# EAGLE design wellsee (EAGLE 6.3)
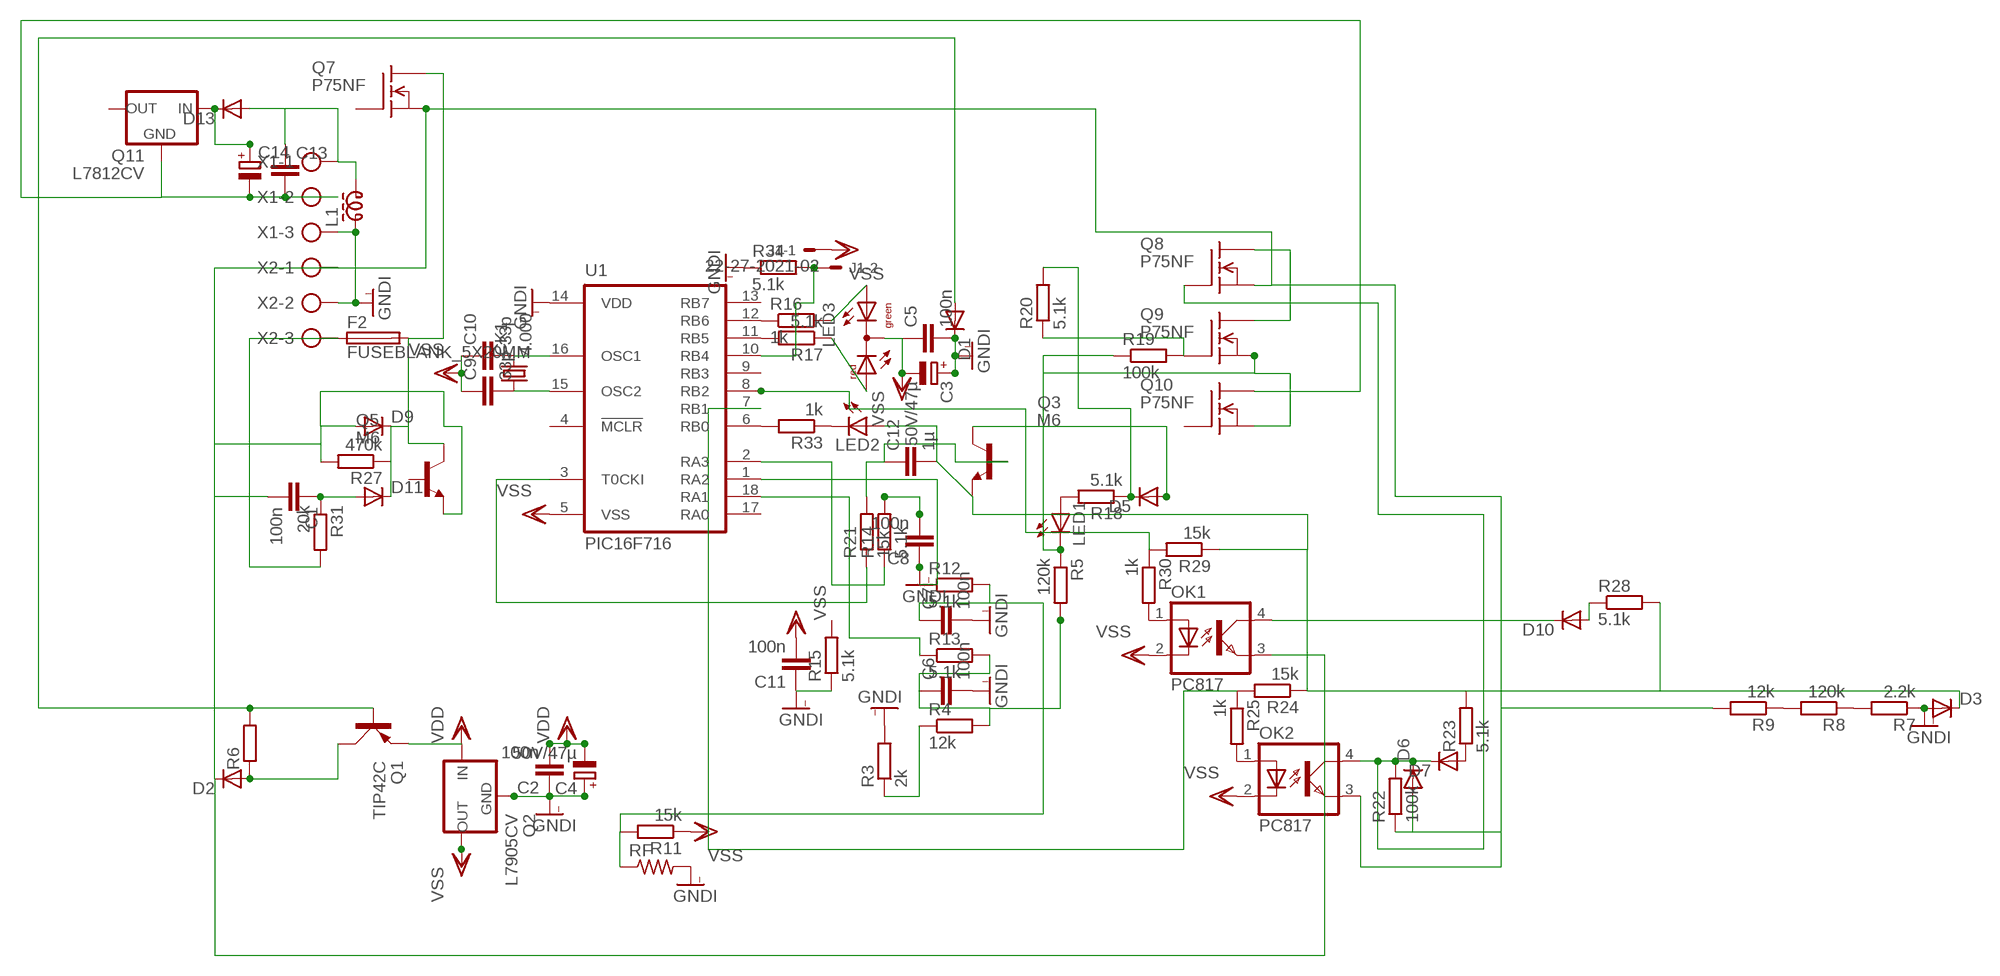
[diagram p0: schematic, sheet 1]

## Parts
C1  100n  C-EUC0805  [C0805]
C2  100n  C-EUC0805  [C0805]
C3  50V/47µ  CPOL-EUE2.5-6  [E2,5-6]
C4  50V/47µ  CPOL-EUE2.5-6  [E2,5-6]
C5  100n  C-EUC0805  [C0805]
C6  100n  C-EUC0805  [C0805]
C7  100n  C-EUC0805  [C0805]
C8  100n  C-EUC0805  [C0805]
C9  33p  C-EUC0805  [C0805]
C10  33p  C-EUC0805  [C0805]
C11  100n  C-EUC0805  [C0805]
C12  1µ  C-EUC0805  [C0805]
C13  C-EU075-032X103  [C075-032X103]
C14  CPOL-EUE5-13  [E5-13]
CK1  4.000  CRYSTALHC49S  [HC49/S]
D1  DIODE-MINIMELF  [MINIMELF]
D2  DIODE-MINIMELF  [MINIMELF]
D3  DIODE-MELF-MLL41  [MELF-MLL41]
D5  DIODE-MINIMELF  [MINIMELF]
D6  DIODE-MINIMELF  [MINIMELF]
D7  DIODE-MINIMELF  [MINIMELF]
D9  DIODE-MINIMELF  [MINIMELF]
D10  DIODE-MINIMELF  [MINIMELF]
D11  DIODE-MELF-MLL41  [MELF-MLL41]
D13  DIODE-MELF-MLL41  [MELF-MLL41]
F2  FUSEBLANK_5X20MM  [FUSE_HOLDER_5X20MM]
J1  22-27-2021-02  [6410-02]
L1  ZD60820512  [ZD6-2W5]
LED1  LED3MM  [LED3MM]
LED2  LED3MM  [LED3MM]
LED3  DUOLED-RG-C  [DUOLED-C-5MM]
OK1  PC817  [DIL04]
OK2  PC817  [DIL04]
Q1  TIP42C  [TO220AV]
Q2  L7905CV  79XXS  [79XXS]
Q3  M6  BC849SMD  [SOT23-BEC]
Q5  M6  BC849SMD  [SOT23-BEC]
Q7  P75NF  SUP75N06-08  [TO220]
Q8  P75NF  SUP75N06-08  [TO220]
Q9  P75NF  SUP75N06-08  [TO220]
Q10  P75NF  SUP75N06-08  [TO220]
Q11  L7812CV  78XXS  [78XXS]
R3  2k  R-EU_R0805  [R0805]
R4  12k  R-EU_R0805  [R0805]
R5  120k  R-EU_R0805  [R0805]
R6  R-EU_0207/5V  [0207/5V]
R7  2.2k  R-EU_R0805  [R0805]
R8  120k  R-EU_R0805  [R0805]
R9  12k  R-EU_R0805  [R0805]
R11  15k  R-EU_R0805  [R0805]
R12  5.1k  R-EU_R0805  [R0805]
R13  5.1k  R-EU_R0805  [R0805]
R14  5.1k  R-EU_R0805  [R0805]
R15  5.1k  R-EU_R0805  [R0805]
R16  1k  R-EU_R0805  [R0805]
R17  5.1k  R-EU_R0805  [R0805]
R18  5.1k  R-EU_R0805  [R0805]
R19  100k  R-EU_R0805  [R0805]
R20  5.1k  R-EU_R0805  [R0805]
R21  15k  R-EU_R0805  [R0805]
R22  100k  R-EU_R0805  [R0805]
R23  5.1k  R-EU_R0805  [R0805]
R24  15k  R-EU_R0805  [R0805]
R25  1k  R-EU_R0805  [R0805]
R27  470k  R-EU_R0805  [R0805]
R28  5.1k  R-EU_R0805  [R0805]
R29  15k  R-EU_R0805  [R0805]
R30  1k  R-EU_R0805  [R0805]
R31  20k  R-EU_R0805  [R0805]
R33  1k  R-EU_R0805  [R0805]
R34  5.1k  R-EU_R0805  [R0805]
RF  R-US_0204/2V  [0204V]
U1  PIC16F716  PIC16C52JW  [DIL18]
X1  AK500/3  [AK500/3]
X2  AK500/3  [AK500/3]

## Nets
GNDI: C2.1 C3.+ C4.+ C5.2 C6.2 C7.2 C8.1 C11.1 D1.C D3.A L1.1 Q2.GND R3.2 R7.1 R15.1 R34.1 RF.2 U1.14(VDD) X1.3 X2.2
N$1: C9.2 CK1.1 U1.15(OSC2)
N$2: C10.2 CK1.2 U1.16(OSC1)
N$3: C7.1 R11.2 R12.2 RF.1
N$5: R33.2 U1.6(RB0)
N$6: LED2.K(C) R33.1
N$7: LED3.AR R17.1
N$8: LED3.AX(AG) R16.2
N$9: R16.1 U1.12(RB6)
N$10: R17.2 U1.11(RB5)
N$11: J1.2 R34.2 U1.10(RB4)
N$12: R14.1 U1.2(RA3)
N$13: R3.1 R4.1
N$14: C6.1 R4.2 R5.2 R13.2
N$15: R13.1 U1.18(RA1)
N$16: LED1.K(C) Q9.3(S) Q10.3(S) R5.1 R19.1
N$17: R21.1 U1.3(T0CKI)
N$18: R12.1 U1.1(RA2)
N$19: C8.2 R14.2
N$20: C12.1 Q3.B R21.2
N$21: C1.2 D2.C D6.A D9.A OK1.3(EMIT) OK2.3(EMIT) Q5.E Q7.3(S) Q8.3(S) R9.2 R22.1 R27.2 X2.1
N$22: C12.2 D3.C LED2.A Q3.E R23.2 R24.1 R28.2 R29.1
N$25: R29.2 R30.1 U1.8(RB2)
N$26: D5.C R18.1 R20.2
N$27: D5.A Q3.C
N$28: OK1.1(A) R30.2
N$29: OK2.1(A) R25.2
N$30: R24.2 R25.1 U1.7(RB1)
N$31: LED1.A R18.2
N$32: D6.C D7.C OK2.4(COL) Q8.1(G) R22.2
N$33: D7.A R23.1
N$34: R8.2 R9.1
N$35: R7.2 R8.1
N$36: Q8.2(D) Q9.2(D)
N$37: D10.C OK1.4(COL)
N$38: D1.A Q1.B R6.2
N$39: D10.A R28.1
N$40: D2.A Q1.C R6.1
N$44: Q9.1(G) R19.2 R20.1
N$48: F2.1 R31.2 X2.3
N$49: D9.C D11.C F2.2 Q5.C Q7.2(D) R27.1
N$51: C13.1 D13.A L1.2 X1.1
N$54: C14.+ D13.C Q11.IN
N$55: C13.2 C14.- Q10.2(D) Q11.GND X1.2
N$56: C1.1 D11.A R31.1
VDD: C2.2 C4.- Q1.E Q2.IN
VSS: C3.- C5.1 C9.1 C10.1 C11.2 J1.1 LED3.C OK1.2(C) OK2.2(C) Q2.OUT R11.1 U1.5(VSS)
Unconnected: Q5.B Q7.1(G) Q10.1(G) Q11.OUT R15.2 U1.4(!MCLR) U1.9(RB3) U1.13(RB7) U1.17(RA0)

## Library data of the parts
C1 C2 C5-C13 = rcl:C-EU: CAPACITOR, European symbol
C3 C4 C14 = rcl:CPOL-EU: POLARIZED CAPACITOR, European symbol
CK1 = crystal:CRYSTAL: CRYSTAL; OC_FARNELL: 1667008; OC_NEWARK: unknown
D1-D3 D5-D7 D9-D11 D13 = diode:DIODE-: DIODE
F2 = fuse:FUSE: Fuse; OC_FARNELL: unknown; OC_NEWARK: unknown
J1 = con-molex:22-?-02: CONNECTOR; OC_FARNELL: unknown; OC_NEWARK: unknown
L1 = inductor-neosid:ZD60820512: WIDE-BAND CHOKE; OC_FARNELL: unknown; OC_NEWARK: unknown
LED1 LED2 = led:LED: LED
LED3 = led:DUOLED-RG-C: DUO LED 2 colors (red/green), 5 mm, round, common Cathode www.ligitek.com or other producers.
OK1 OK2 = optocoupler:PC817: SHARP OPTO COUPLER; MPN: PC817X4J000F; OC_FARNELL: 9707727; OC_NEWARK: 97K7059
Q1 = transistor-power:TIP42C: PNP TRANSISTOR
Q2 = v-reg:79XXS: VOLTAGE REGULATOR
Q3 Q5 = transistor-npn:BC849*: NPN Transistor
Q7-Q10 = transistor-fet:SUP75N06-08: N-Channel Enhancement MOSFET 60V; 75A; 0,008Ohm
Q11 = v-reg:78XXS: VOLTAGE REGULATOR
R3-R9 R11-R25 R27-R31 R33 R34 = rcl:R-EU_: RESISTOR, European symbol
RF = rcl:R-US_: RESISTOR, American symbol
U1 = microchip:PIC16C52: MICROCONTROLLER; OC_FARNELL: unknown; OC_NEWARK: unknown
X1 X2 = con-ptr500:AK500/3: CONNECTOR; OC_FARNELL: unknown; OC_NEWARK: unknown

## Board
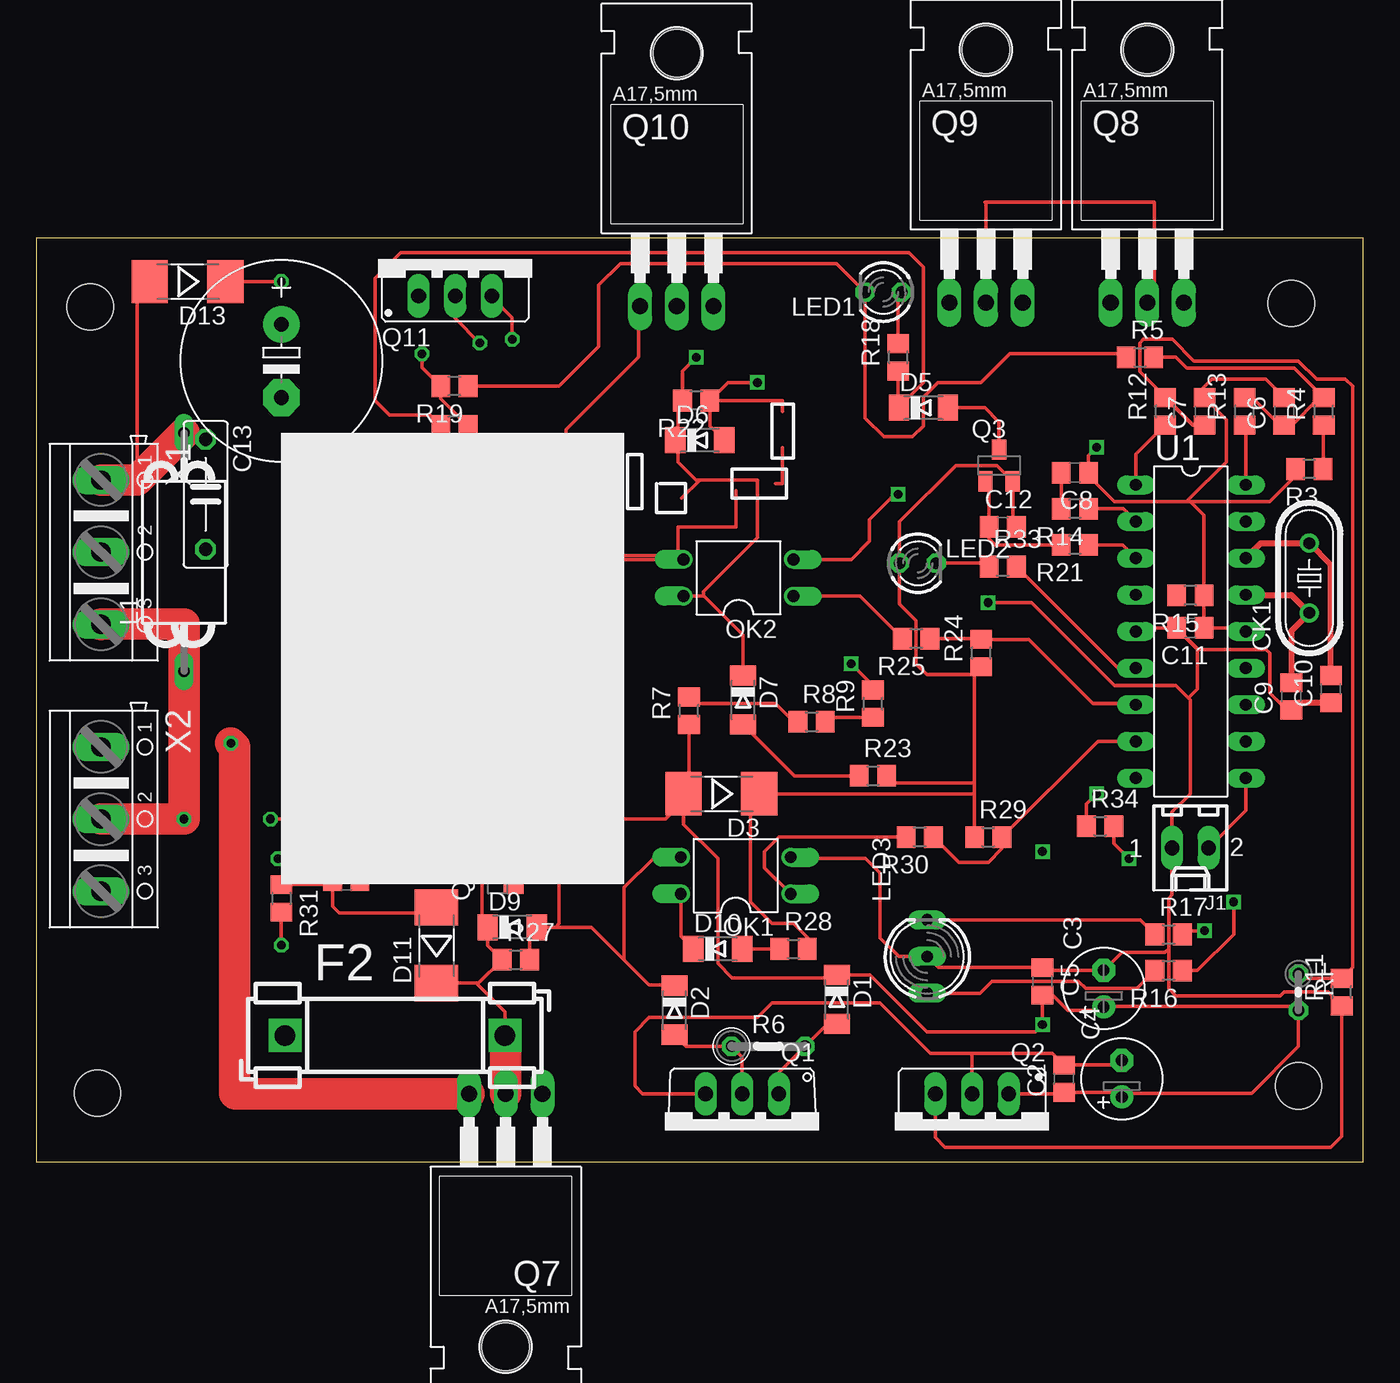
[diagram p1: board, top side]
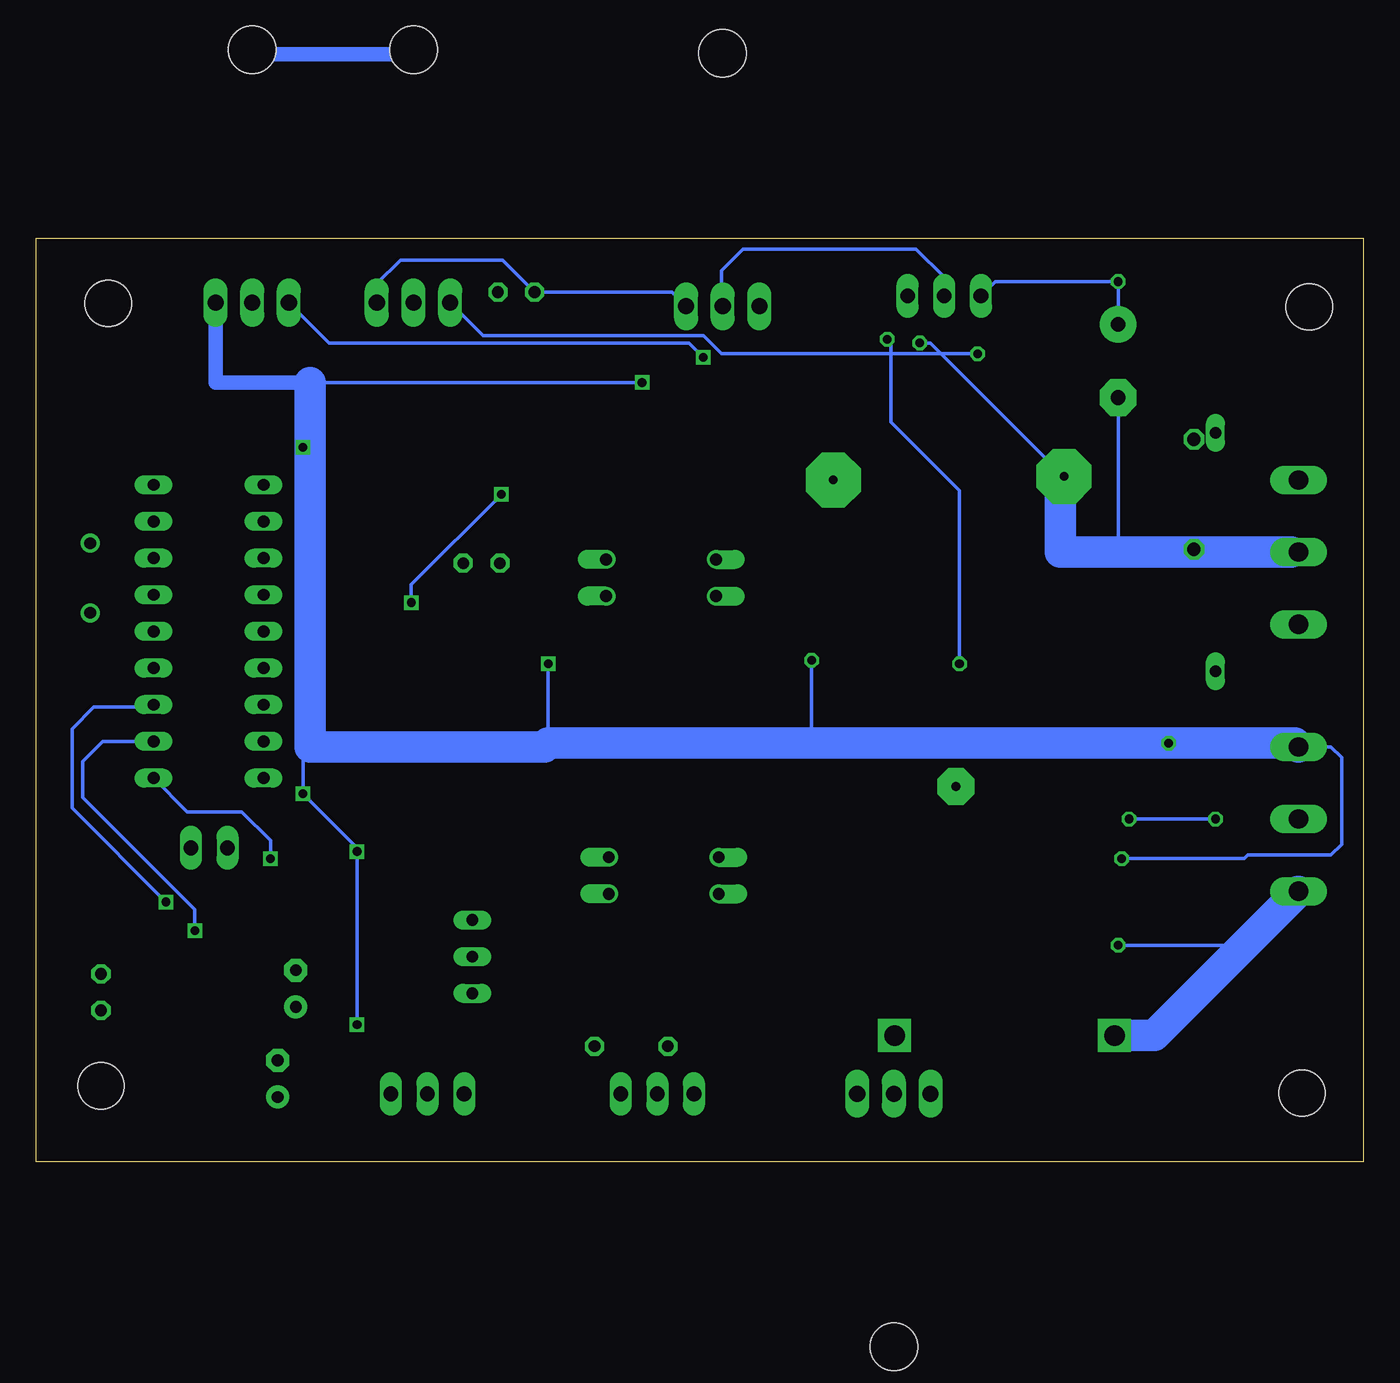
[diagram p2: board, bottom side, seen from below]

Size 92 x 64 mm. Coordinates in mm from the lower left corner, seen from the top.
Outline: 0,0 92,0 92,64 0,64 0,0
Copper layers (1*16): Top 0.035mm / dielectric 1.5mm / Bottom 0.035mm
Design rules "default": minimum track width 10mil, minimum drill 24mil, track to track 8mil, track to pad 8mil, pad to pad 8mil, via to via 8mil, smd to smd 8mil, copper to edge 40mil, drill to drill 8mil, minimum pad ring 10mil, minimum via ring 8mil, stop-mask expansion 4mil, vias tented up to drill 0mil, thermal gap 10mil
Holes 3.2 mm at 3.75,59.25 87,59.5 87.5,5.25 4.25,4.75

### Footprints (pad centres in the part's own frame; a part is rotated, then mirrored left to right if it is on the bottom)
C0805 = smd 1.3 x 1.5: 1 -0.95,0; 2 0.95,0
E2,5-6 = drill 0.813 pad 1.6: + -1.27,0 | drill 0.813 pad 1.6 octagon: - 1.27,0
C075-032X103 = drill 0.914 octagon: 1 -3.81,0; 2 3.81,0
E5-13 = drill 1.016 pad 2.54: + -2.54,0 | drill 1.016 pad 2.54 octagon: - 2.54,0
HC49/S = drill 0.813: 1 -2.413,0; 2 2.413,0
MINIMELF = smd 1.4 x 1.8: A 1.7,0; C -1.7,0
MELF-MLL41 = smd 2.5 x 3: A 2.625,0; C -2.625,0
FUSE_HOLDER_5X20MM = drill 1.422 pad 2.286 square: 1 0,0; 2 15.24,0
6410-02 = drill 1.016 long: 1 1.27,0; 2 -1.27,0
ZD6-2W5 = drill 0.8 long: 1 -8.255,0; 2 8.255,0
LED3MM = drill 0.813 octagon: A -1.27,0; K 1.27,0
DUOLED-C-5MM = drill 0.813 long: AR 2.54,0; AX -2.54,0; C 0,0
DIL04 = drill 0.813 offset: 1 -1.27,-3.81; 2 1.27,-3.81; 3 1.27,3.81; 4 -1.27,3.81
TO220AV = drill 1.016 long: B -2.54,-2.54; C 0,-2.54; E 2.54,-2.54
79XXS = drill 1.016 long: GND -2.54,-2.54; IN 0,-2.54; OUT 2.54,-2.54
SOT23-BEC = smd 1 x 1.4: B -0.95,-1.1; C 0,1.1; E 0.95,-1.1
TO220 = drill 1.118 long: 1 -2.54,-6.35; 2 0,-6.35; 3 2.54,-6.35 | hole 3.302: 0,11.176
78XXS = drill 1.016 long: GND 0,-2.54; IN -2.54,-2.54; OUT 2.54,-2.54
R0805 = smd 1.3 x 1.5: 1 -0.95,0; 2 0.95,0
0207/5V = drill 0.813 octagon: 1 -2.54,0; 2 2.54,0
0204V = drill 0.813 octagon: 1 -1.27,0; 2 1.27,0
DIL18 = drill 0.813 long: 1 -10.16,-3.81; 2 -7.62,-3.81; 3 -5.08,-3.81; 4 -2.54,-3.81; 5 0,-3.81; 6 2.54,-3.81; 7 5.08,-3.81; 8 7.62,-3.81; 9 10.16,-3.81; 10 10.16,3.81; 11 7.62,3.81; 12 5.08,3.81; 13 2.54,3.81; 14 0,3.81; 15 -2.54,3.81; 16 -5.08,3.81; 17 -7.62,3.81; 18 -10.16,3.81
AK500/3 = drill 1.321 long: 1 -5.004,0; 2 0,0; 3 5.004,0

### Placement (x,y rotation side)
C1  21.5,19.5 0 top
C2  71.25,5.75 90 top
C3  74,12 90 top
C4  75.25,5.75 90 top
C5  69.75,12.5 270 top
C6  86.5,52 90 top
C7  81,52 90 top
C8  72,47.75 180 top
C9  87,32.25 90 top
C10  89.75,32.75 90 top
C11  80,37 180 top
C12  67,44 0 top
C13  11.75,46.25 270 top
C14  17,55.5 270 top
CK1  88.25,40.45 90 top
D1  55.5,11.25 270 top
D2  44.25,10.5 270 top
D3  47.5,25.5 180 top
D5  61.5,52.25 0 top
D6  46,50 0 top
D7  49,32 270 top
D9  33,16.25 0 top
D10  47.25,14.75 0 top
D11  27.75,15 90 top
D13  10.5,61 180 top
F2  17.25,8.75 0 top
J1  80,21.75 180 top
L1  10.25,42.25 90 top
LED1  58.72,60.27 180 top
LED2  61.12,41.48 0 top
LED3  61.77,14.21 90 top
OK1  48.5,19.83 90 top
OK2  48.68,40.47 90 top
Q1  48.94,2.16 180 top
Q2  64.87,2.16 180 top
Q3  66.75,48.25 0 top
Q5  32,20 90 top
Q7  32.55,-1.64 180 top
Q8  77.02,65.89 0 top
Q9  65.84,65.89 0 top
Q10  44.41,65.64 0 top
Q11  29.05,62.54 0 top
R3  88.25,48 180 top
R4  89.25,52 90 top
R5  76.5,55.75 0 top
R6  50.75,8 0 top
R7  45.25,31.25 90 top
R8  53.75,30.5 0 top
R9  58,31.75 90 top
R11  90.5,11.75 90 top
R12  78.25,52 90 top
R13  83.75,52 90 top
R14  72,45.25 180 top
R15  80,39.25 180 top
R16  78.5,13.25 180 top
R17  78.5,15.75 0 top
R18  59.75,55.75 90 top
R19  29,53.75 180 top
R20  29,51 180 top
R21  72,42.75 180 top
R22  45.75,52.75 180 top
R23  58,26.75 0 top
R24  65.5,35.25 90 top
R25  61,36.25 180 top
R27  33.25,14 0 top
R28  52.5,14.75 0 top
R29  66,22.5 0 top
R30  61.25,22.5 180 top
R31  17,18.25 270 top
R33  67,41.25 0 top
R34  73.75,23.25 0 top
RF  87.5,11.75 270 top
U1  80.04,36.75 270 top
X1  4.5,42.25 270 top
X2  4.5,23.75 270 top

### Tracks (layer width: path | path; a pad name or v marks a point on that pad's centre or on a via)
GNDI  (via drill 0.6)
  Top 0.254: Q2.GND 71.15,4.7 C2.1 74.93,4.8 C4.+ 75.52,4.75 84.25,4.75 87.5,8 RF.2 87.23,10.75 74,10.75 73.75,10.5 | 73.75,10.5 73.77,10.5 C3.+ | 73.75,10.5 71.5,10.5 70.45,11.55 C5.2 v69.75,9.5 69.25,9 61.75,9 57.8,12.95 D1.C 55.3,12.75 48.25,12.75 47.25,13.75 47.25,21 44.88,23.38 44.88,25 | R34.1 72.8,24.8 v73.5,25.5 | C6.2 86.5,53 85.25,54.25 81.5,54.25 80.75,53.5 80.75,53.2 C7.2 82.5,51.45 82.5,48.5 79.88,45.88 | v73.5,49.5 72.95,48.95 C8.1 72.95,47.55 74.75,45.75 79.75,45.75 | 79.75,45.75 79.88,45.88 | R3.2 87.3,47.55 85.5,45.75 79.75,45.75 | 79.88,45.88 80.95,44.8 R15.1 C11.1 83.6,37 U1.14 | R7.1 45.25,25.88 D3.A 44.88,25 | v16.25,23.75 43.62,23.75 44.88,25
  Top 2.184: X2.2 v10.25,23.75 L1.1 | L1.1 10.25,37.25 9.5,37.25 | 9.5,37.25 X1.3 | L1.1 10.25,36.5 9.5,37.25
  Bottom 0.254: v69.75,9.5 v69.75,21.5 69.75,21.75 v73.5,25.5 v73.5,49.5 | v10.25,23.75 v16.25,23.75
N$1
  Top 0.406: U1.15 87,39.29 CK1.1 87,36.79 C9.2
N$2
  Top 0.406: U1.16 84.88,42.86 CK1.2 89.75,41.36 C10.2
N$3
  Top 0.254: R12.2 80.15,51.05 C7.1 80.2,51.05 76.5,54.75 76.5,56.75 76.75,57 78.75,57 80.25,55.5 87.5,55.5 88.75,54.25 90.75,54.25 91.25,53.75 91.25,13.45 R11.2 87.82,12.7 RF.1
N$4
  Top 0.254: 86.75,31.5 86.5,31.5
N$5
  Top 0.254: U1.6 74.99,34.21 R33.2
N$6
  Top 0.254: LED2.K 65.82,41.48 R33.1
N$7
  Top 0.254: LED3.AR 76.55,16.75 R17.1
N$8
  Top 0.254: LED3.AX 65.42,11.67 66.25,12.5 72.25,12.5 72.75,12 76.3,12 R16.2
N$9  (via drill 0.6)
  Top 0.254: R16.1 80.5,13.25 83,15.75 v83,18
  Bottom 0.254: v83,18 89.5,24.5 89.5,30 88,31.5 84.02,31.5 U1.12
N$10  (via drill 0.6)
  Top 0.254: v81,16 79.7,16 R17.2
  Bottom 0.254: U1.11 87.37,29.13 88.75,27.75 88.75,25.25 81,17.5 v81,16
N$11  (via drill 0.6)
  Top 0.254: J1.2 83.85,24.33 U1.10 | R34.2 74.7,22.05 v75.75,21
  Bottom 0.254: v75.75,21 75.75,22.25 77.75,24.25 81.51,24.25 U1.10
N$12
  Top 0.254: R14.1 75.35,45.25 U1.2
N$13
  Top 0.254: R3.1 89.2,51 R4.1
N$14
  Top 0.254: R13.2 83.95,52.75 84.5,52.75 86.2,51.05 C6.1 86.55,51 87,51 88.95,52.95 R4.2 87.2,55 79.75,55 79,55.75 R5.2
N$15
  Top 0.254: U1.18 83.85,50.95 R13.1
N$16
  Top 0.254: R5.1 75.3,56 67.5,56 65.5,54 62.5,54 61.5,53 61.5,51 60.75,50.25 58.75,50.25 57.45,51.55 LED1.K 55.47,62.25 40.5,62.25 39,60.75 39,56.5 36.25,53.75 R19.1
  Bottom 0.254: Q10.3 47.93,60.27 LED1.K 59.68,62.5 66.75,62.5 68.38,60.87 Q9.3
N$17
  Top 0.254: R21.1 75.31,42.75 U1.3
N$18
  Top 0.254: U1.1 76.23,49.03 R12.1
N$19
  Top 0.254: R14.2 C8.2
N$20
  Top 0.254: R21.2 66.5,42.75 66.05,43.2 C12.1 66.05,46.9 Q3.B
N$21  (via drill 0.6)
  Top 0.254: OK1.3 42.85,21.1 40.75,19 40.75,14 | 40.75,14 42.5,12.25 44.2,12.25 D2.C | D9.A 34.2,15.75 R27.2 34.2,15.95 34.5,16.25 D9.A | D9.A 36,16.25 | 36,16.25 38.5,16.25 40.75,14 | 35.8,20.95 Q5.E 32.05,22 32,22 | 35.8,20.95 36.25,20.5 36.25,16.5 36,16.25 | C1.2 22.45,19.95 24.5,22 | v50,54 47.95,54 R22.1 46.7,51 D6.A | R9.2 58,33 v56.5,34.5 | 35.8,20.95 35.75,21 33,21 32,22 | 32,22 24.5,22 | 24.5,22 21.5,22 20.5,21 v16.75,21 | OK2.3 38.51,41.74 38.25,42 v38.25,34.75
  Top 2.184: Q7.3 13.79,4.71 13.75,4.75 13.75,28.75 v13.5,29
  Bottom 0.254: 73,54 v50,54 | v56.5,34.5 56.5,29 56.75,28.75 | v16.75,21 8.25,21 8,21.25 2.25,21.25 1.5,22 1.5,28 2.25,28.75 X2.1 | v38.25,34.75 38.25,29
  Bottom 1.016: 73,54 79.56,54 Q8.3
  Bottom 2.184: 56.75,28.75 73,28.75 73,54 | 56.5,29 38.25,29 v13.5,29 4.75,29 X2.1
N$22
  Top 0.254: C12.2 67.7,44.25 Q3.E 66.6,48.25 63.75,48.25 59.85,44.35 LED2.A 59.85,38.65 61,37.5 61,34.5 61.75,33.75 64.95,33.75 65.05,33.85 | 65.05,26.2 65.05,33.85 | 65.05,33.85 R24.1 | R29.1 65.05,25.5 | 65.05,25.5 65.05,26.2 | 65.05,26.2 65,26.25 59.45,26.25 R23.2 | 65.05,25.5 D3.C 49.5,24.88 49.5,18 51,16.5 52.5,16.5 53.45,15.55 R28.2
N$23
  Bottom 1.016: 65.5,76.75 77.25,76.75
N$24
  Bottom 1.016: 44.25,77 44.75,77
N$25
  Top 0.254: U1.8 73.58,29.13 R29.2 66.95,21.7 66,20.75 63.95,20.75 R30.1
N$26
  Top 0.254: 59.8,54.75 R18.1 59.75,52.3 D5.C 59.8,52.3 61.5,54 61.5,62 60.5,63 25.25,63 23.5,61.25 23.5,52.75 24.5,51.75 27.3,51.75 R20.2
N$27
  Top 0.254: Q3.C 66.75,51.25 65.75,52.25 D5.A
N$28
  Top 0.254: R30.2 51.5,22.5 50.5,21.5 50.5,20.37 OK1.1
N$29
  Top 0.254: OK2.1 57.1,39.2 R25.2
N$30
  Top 0.254: R25.1 65.45,36.25 R24.2 68.8,36.2 73.25,31.75 76.15,31.75 U1.7
N$31
  Top 0.254: R18.2 59.75,60.03 LED1.A
N$32  (via drill 0.6)
  Top 0.254: D7.C 49,36.5 46.25,39.25 | 46.25,39.25 46.25,39.5 50,43.25 50,47.25 46,47.25 | 44.75,46 46,47.25 | 46,47.25 45.75,47.25 44.5,48.5 44.5,49.8 D6.C 44.3,50.8 44.5,51 44.5,52.45 R22.2 44.8,54.8 v45.75,55.75 | OK2.4 46.2,39.2 46.25,39.25
  Bottom 0.254: v45.75,55.75 46.75,56.75 71.69,56.75 Q8.1
N$33
  Top 0.254: R23.1 52.55,26.75 D7.A
N$34
  Top 0.254: R9.1 55,30.8 R8.2
N$35
  Top 0.254: R8.1 52.5,30.5 51.25,31.75 45.7,31.75 R7.2
N$36
  Top 0.254: Q9.2 65.84,66.41 65.75,66.5 77.5,66.5 77.5,60.02 Q8.2
N$37
  Top 0.254: OK1.4 44.69,15.61 D10.C
N$38
  Top 0.254: Q1.B 51.48,6.19 R6.2 54.84,9.55 D1.A
N$39
  Top 0.254: D10.A R28.1
N$40
  Top 0.254: Q1.C 48.94,7.27 R6.1 45.05,8 D2.A
N$41  (via drill 0.6 pad 3.81)
  Top 0.254: v36.75,47.25 36.75,50.75 41.75,55.75 41.75,59.25 42,59.5 41.75,59.5
N$42  (via drill 0.6 pad 3.81)
  other vias: 20.75,47.5
N$43  (via drill 0.6 pad 2.54)
  other vias: 28.25,26
N$44  (via drill 0.6)
  Top 0.254: v26.75,56 26.75,55.05 R19.2 28.05,52.9 R20.1
  Bottom 0.254: Q9.1 61.01,57.25 45.75,57.25 44.5,56 v26.75,56
N$45
  Top 0.254: 51.75,52 51.75,52.75 46.75,52.75 | 46.75,53 46.75,52.75 | 46.75,52.75 46.5,52.75
N$46
  Top 0.254: 51.75,49.5 51.75,47 51.25,47
N$47
  Top 0.254: 48.5,46.5 48.5,44 44.5,44 44.5,42 38.25,42 38.25,35
N$48  (via drill 0.6)
  Top 0.254: R31.2 v17,15
  Bottom 0.254: v17,15 8.25,15 7.5,15.75
  Bottom 2.184: F2.1 14.5,8.75 7.5,15.75 X2.3
N$49
  Top 0.254: 30.5,12.38 30.68,12.38 R27.1 31.3,15 D9.C 30.9,16.65 Q5.C | F2.2 32.49,10.38 30.5,12.38 | D11.C 30.5,12.38
  Top 2.184: Q7.2 32.55,8.69 F2.2
N$51
  Top 0.254: 7,47.25 7,60.12 D13.A | C13.1 10.7,50.06 L1.2
  Top 2.184: X1.1 7,47.25 L1.2
N$52
  Bottom 2.184: 5,42.25 21,42.25 21,47.5 | 21,47.75 21,47.5 | 21,47.5 20.75,47.5 20.75,47.75
N$54  (via drill 0.6)
  Top 0.254: D13.C v17,61
  Bottom 0.254: Q11.IN 25.51,61 v17,61 C14.+
N$55  (via drill 0.6)
  Top 0.254: Q11.GND 29.05,58.45 v30.75,56.75
  Bottom 0.254: Q11.GND 29.05,61.3 31,63.25 43,63.25 44.5,61.75 44.5,59.38 Q10.2 | v30.75,56.75 30,56.75 20.75,47.5 20.75,42.25 16.75,42.25 | 16.75,42.25 14,42.25 | 14,42.25 X1.2 | C14.- 17,42.5 16.75,42.25 | C13.2 13.81,42.44 14,42.25
N$56
  Top 0.254: D11.A 27.38,17.25 21,17.25 20.55,17.7 C1.1 20.25,19.2 R31.1
N$58  (via drill 0.6)
  Top 0.254: 28,25.75 v28,34.5 | v33,57 33,58.5 31.75,59.75
  Bottom 0.254: v28,34.5 28,46.5 32.75,51.25 32.75,56.75 v33,57
VDD
  Top 0.254: Q1.E 42.05,4.7 41.5,5.25 41.5,9 42.5,10 50,10 51,11 58.5,11 62,7.5 64.75,7.5 | 64.75,7.5 70.45,7.5 C2.2 74.93,6.7 C4.- | Q2.IN 64.87,7.38 64.75,7.5
VSS  (via drill 0.6)
  Top 0.254: C9.1 86.7,31.3 85.5,32.5 85.5,35.25 85.25,35.5 80.55,35.5 C11.2 79,37 | 76.5,37 76.48,37 U1.5 76.25,36.75 76.5,37 | 79.88,32.12 80,32 80,25.5 78.73,24.23 J1.1 78.73,18.48 78.5,18.25 78.5,14.75 | 79.88,32.12 79,33 74.75,33 69,38.75 v66,38.75 | 76.5,37 79,37 | 79,37 80.5,35.5 80.5,32.75 79.88,32.12 | 78.5,14.75 78.5,12 79,11.5 86.25,11.5 86.5,11.75 89.55,11.75 R11.1 90.5,1.75 89.75,1 63,1 62.33,1.67 Q2.OUT | 78.5,14.75 78.25,14.5 75.25,14.5 74.02,13.27 C3.- 69.93,13.27 C5.1 62.53,13.45 LED3.C 59.79,14.21 58.5,15.5 58.5,20 57.5,21 52.41,21 OK1.2 | v59.75,46.25 59.5,46.25 57.75,44.5 57.75,43 56.5,41.75 OK2.2
  Top 0.406: C10.1 87.5,31.8 C9.1
  Bottom 0.254: v66,38.75 66,40 v59.75,46.25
